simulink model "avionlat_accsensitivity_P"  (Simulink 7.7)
settings: Solver=ode45  StartTime=0.0  StopTime=10.0  RelTol=1e-3
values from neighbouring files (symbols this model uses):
  A = tf([5],[1 5])    [demo_section_2_5.m]
  D = D(index12,index12)    [cor2tfg.m]    (also in cor2obr.m = D(index132,index132))
undefined symbols (not defined in the file or in its folder): B, C

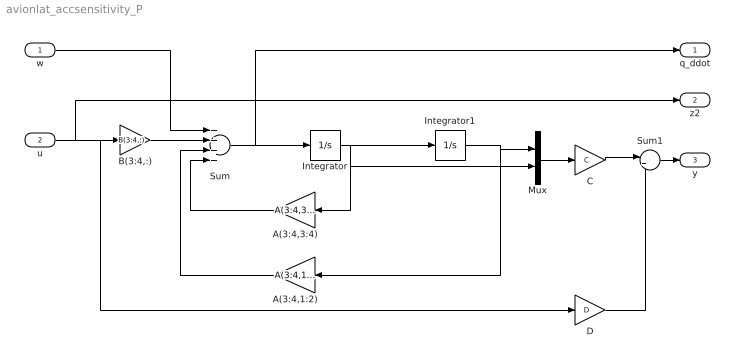
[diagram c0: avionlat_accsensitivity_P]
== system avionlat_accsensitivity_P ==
  w : Inport  PortDimensions=2
  u : Inport  Port=2  PortDimensions=2
  A(3:4,1:2) : Gain  Gain=A(3:4,1:2)  Multiplication=Matrix(K*u)
  A(3:4,3:4) : Gain  Gain=A(3:4,3:4)  Multiplication=Matrix(K*u)
  B(3:4,:) : Gain  Gain=B(3:4,:)  Multiplication=Matrix(K*u)
  C : Gain  Gain=C  Multiplication=Matrix(K*u)
  D : Gain  Gain=D  Multiplication=Matrix(K*u)
  Integrator : Integrator
  Integrator1 : Integrator
  Mux : Mux  Inputs=2
  Sum : Sum  Inputs=++++
  Sum1 : Sum  Inputs=|++
  q_ddot : Outport
  z2 : Outport  Port=2
  y : Outport  Port=3
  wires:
  Sum/1 -> Integrator/1, q_ddot/1
  Integrator/1 -> Integrator1/1, A(3:4,3:4)/1, Mux/2
  Integrator1/1 -> A(3:4,1:2)/1, Mux/1
  A(3:4,3:4)/1 -> Sum/4
  A(3:4,1:2)/1 -> Sum/3
  w/1 -> Sum/1
  B(3:4,:)/1 -> Sum/2
  Mux/1 -> C/1
  C/1 -> Sum1/1
  D/1 -> Sum1/2
  u/1 -> B(3:4,:)/1, D/1, z2/1
  Sum1/1 -> y/1
